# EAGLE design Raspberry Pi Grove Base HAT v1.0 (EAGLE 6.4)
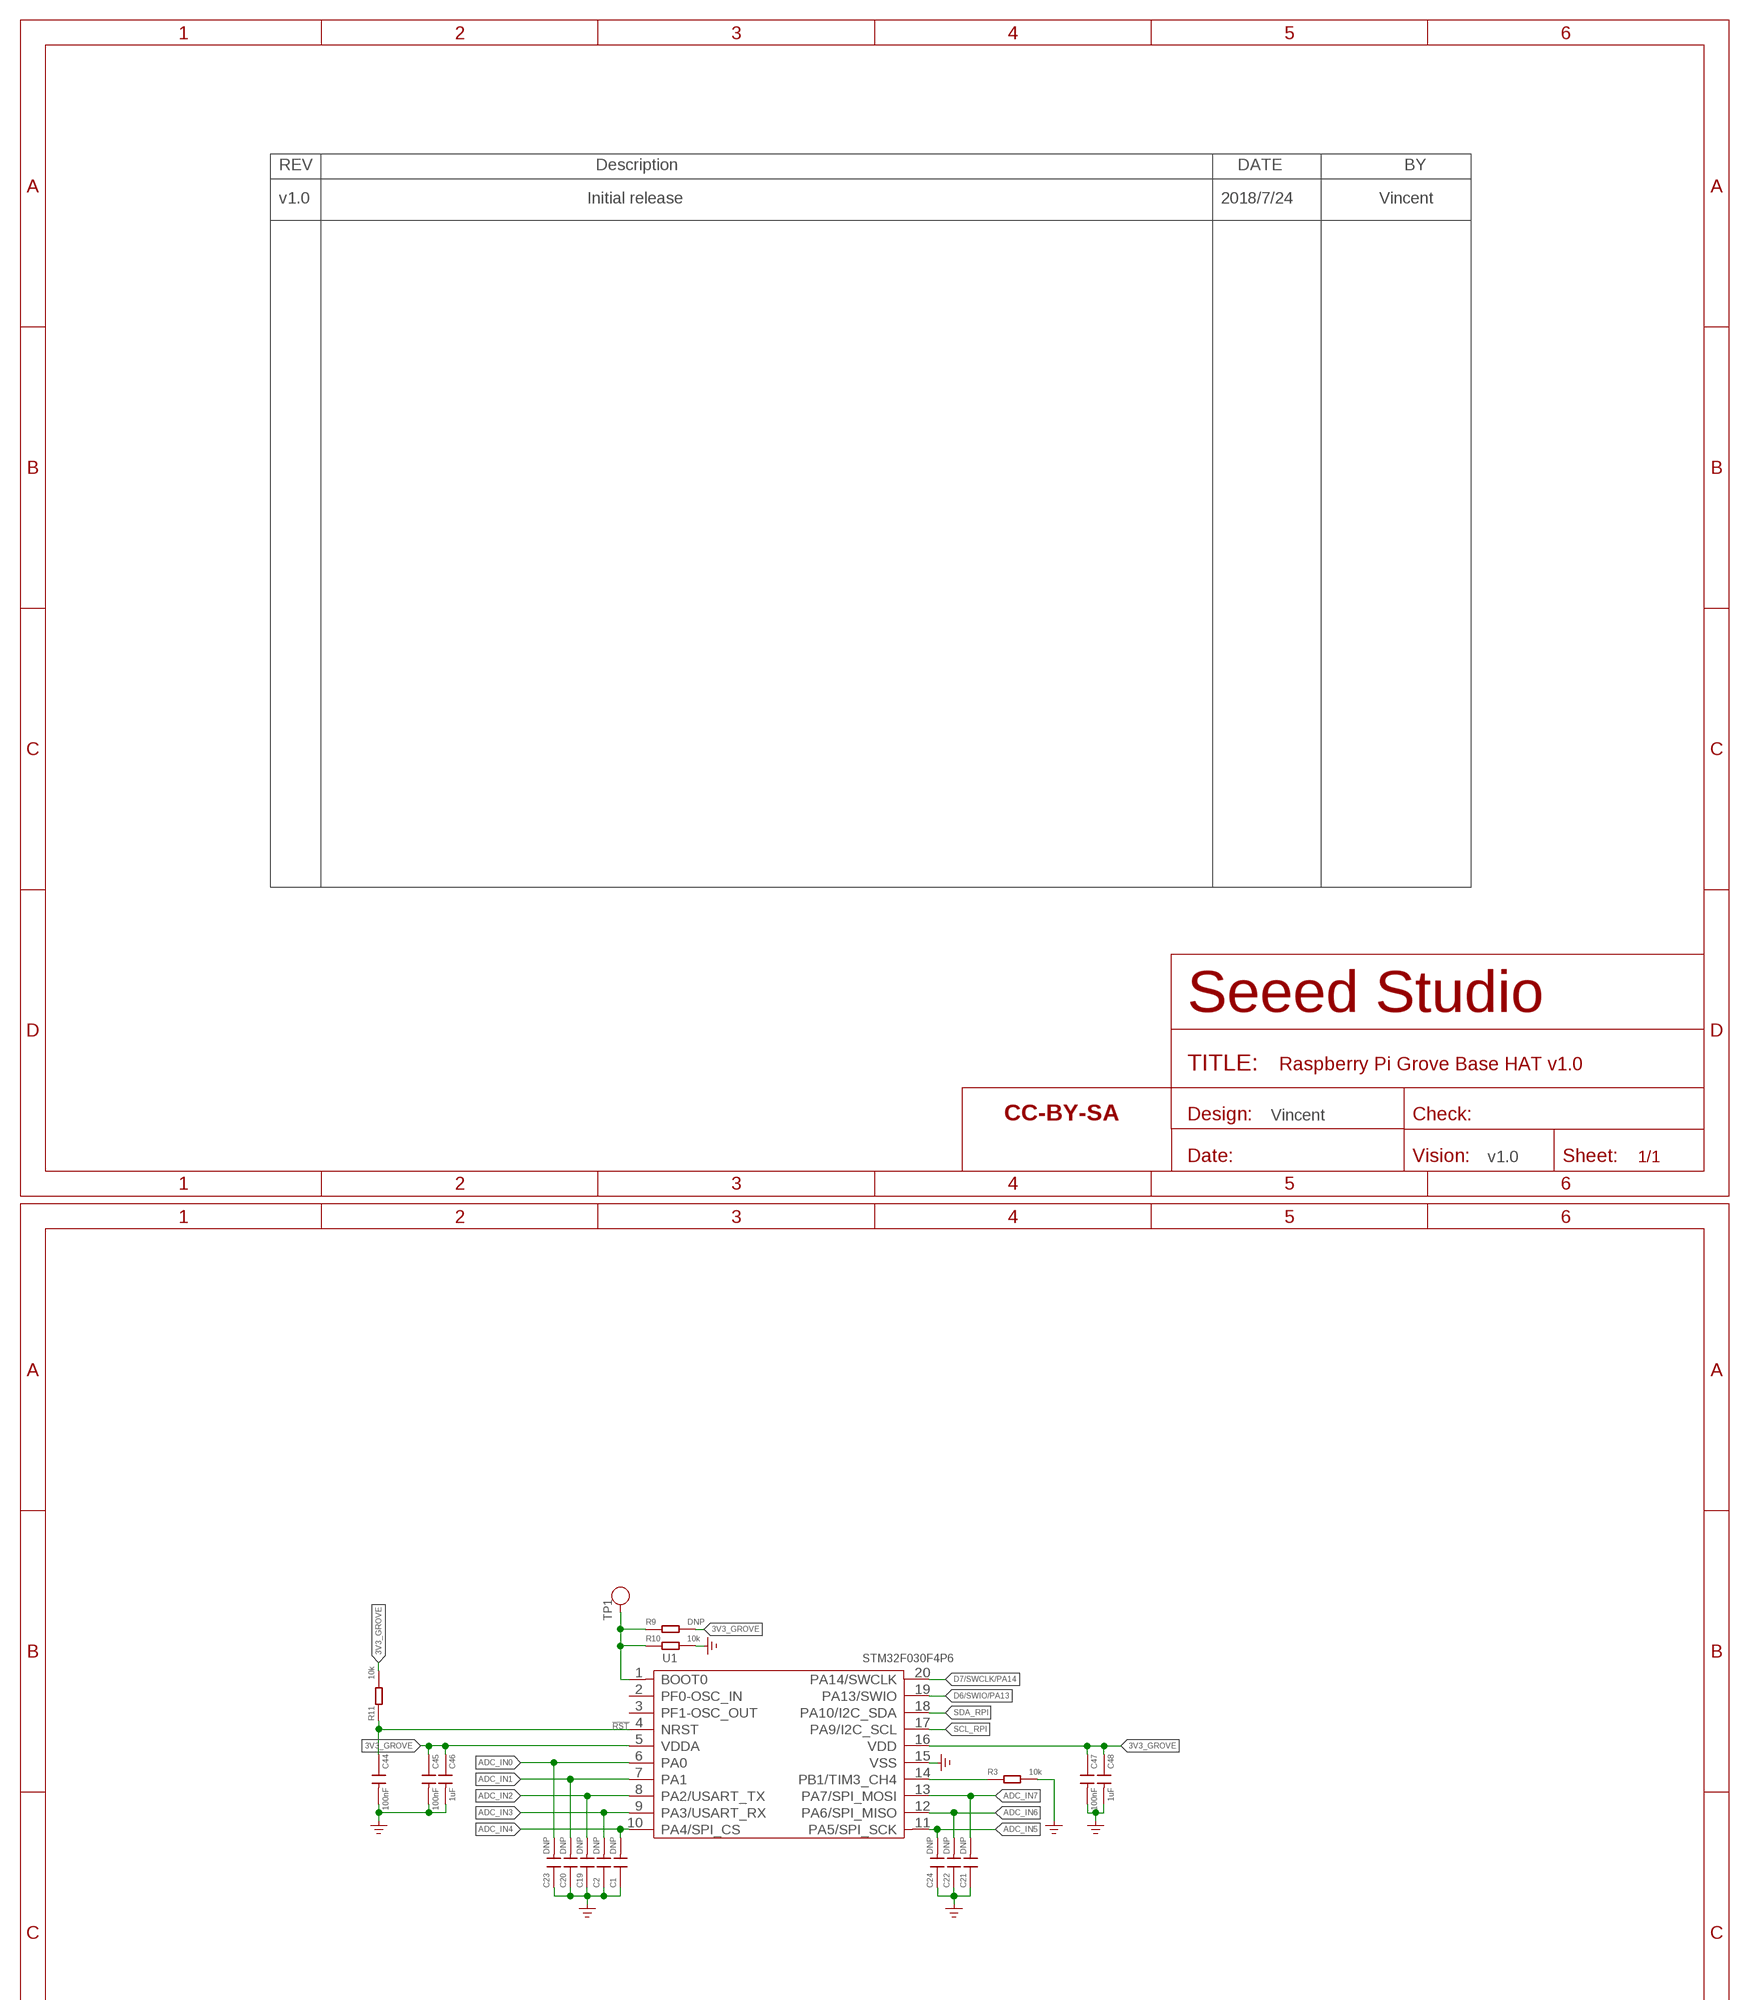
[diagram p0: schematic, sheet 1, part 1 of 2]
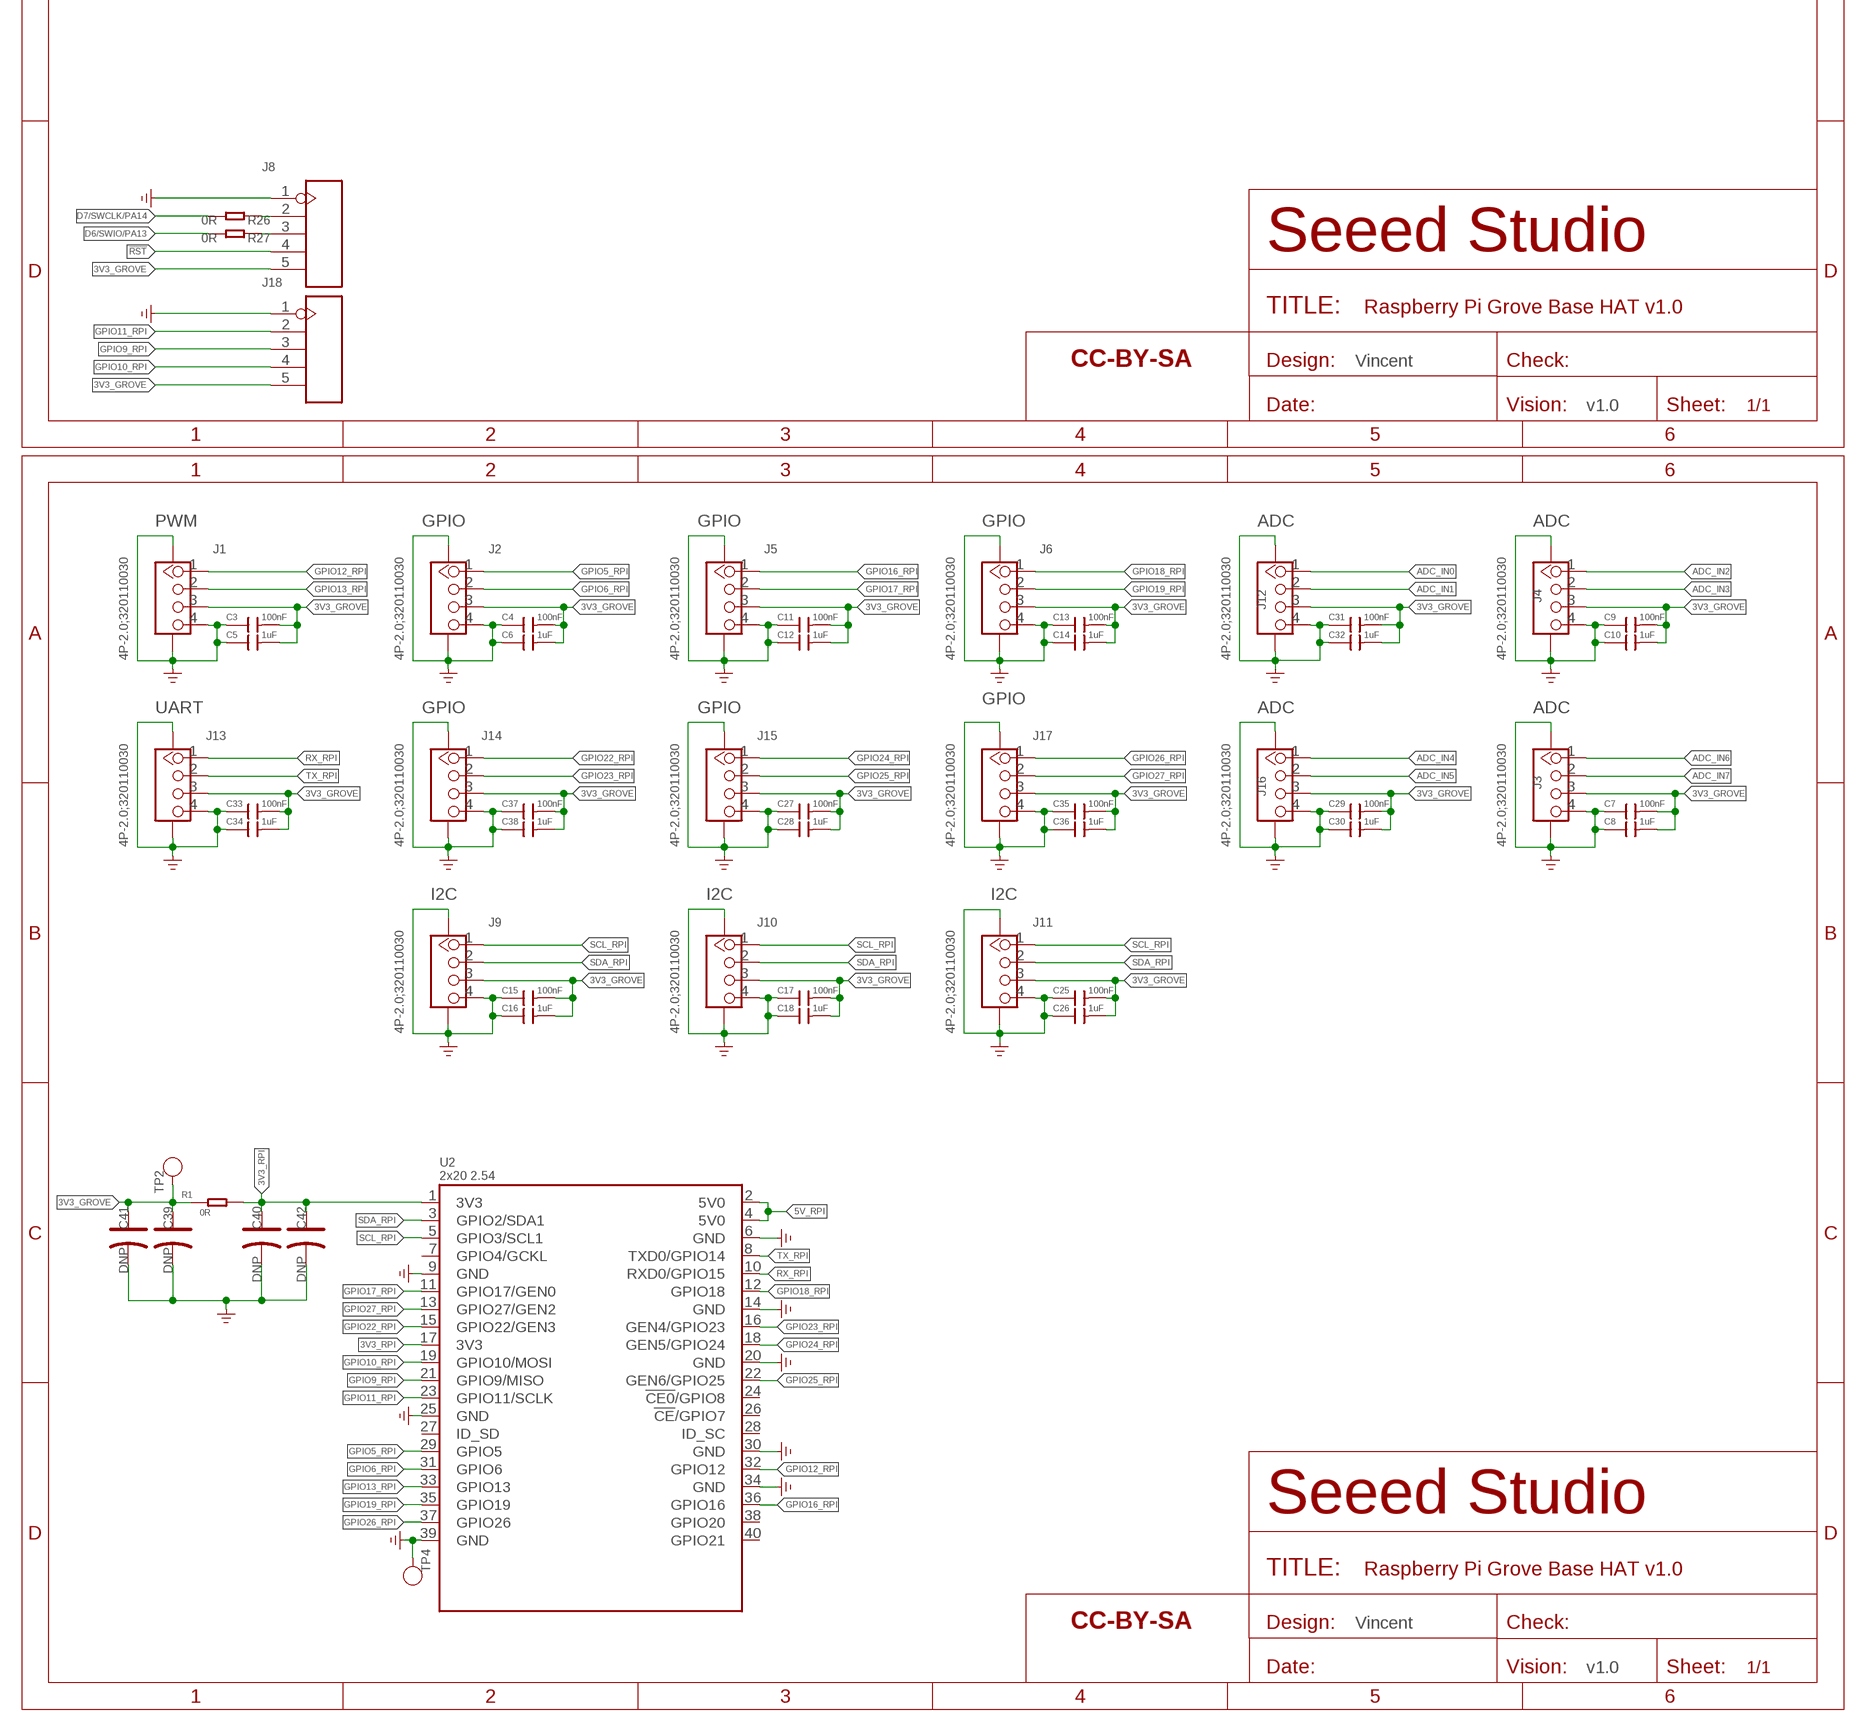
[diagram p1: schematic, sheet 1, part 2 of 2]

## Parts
C1  DNP  C-0603  [C0603]
C2  DNP  C-0603  [C0603]
C3  100nF  C-0603  [C0603]
C4  100nF  C-0603  [C0603]
C5  1uF  C-0603  [C0603]
C6  1uF  C-0603  [C0603]
C7  100nF  C-0603  [C0603]
C8  1uF  C-0603  [C0603]
C9  100nF  C-0603  [C0603]
C10  1uF  C-0603  [C0603]
C11  100nF  C-0603  [C0603]
C12  1uF  C-0603  [C0603]
C13  100nF  C-0603  [C0603]
C14  1uF  C-0603  [C0603]
C15  100nF  C-0603  [C0603]
C16  1uF  C-0603  [C0603]
C17  100nF  C-0603  [C0603]
C18  1uF  C-0603  [C0603]
C19  DNP  C-0603  [C0603]
C20  DNP  C-0603  [C0603]
C21  DNP  C-0603  [C0603]
C22  DNP  C-0603  [C0603]
C23  DNP  C-0603  [C0603]
C24  DNP  C-0603  [C0603]
C25  100nF  C-0603  [C0603]
C26  1uF  C-0603  [C0603]
C27  100nF  C-0603  [C0603]
C28  1uF  C-0603  [C0603]
C29  100nF  C-0603  [C0603]
C30  1uF  C-0603  [C0603]
C31  100nF  C-0603  [C0603]
C32  1uF  C-0603  [C0603]
C33  100nF  C-0603  [C0603]
C34  1uF  C-0603  [C0603]
C35  100nF  C-0603  [C0603]
C36  1uF  C-0603  [C0603]
C37  100nF  C-0603  [C0603]
C38  1uF  C-0603  [C0603]
C39  DNP  CAP-POLAR-AVX-B  [AVX-B]
C40  DNP  CAP-POLAR-AVX-B  [AVX-B]
C41  DNP  CAP-POLAR-AVX-B  [AVX-B]
C42  DNP  CAP-POLAR-AVX-B  [AVX-B]
C44  100nF  C-0603  [C0603]
C45  100nF  C-0603  [C0603]
C46  1uF  C-0603  [C0603]
C47  100nF  C-0603  [C0603]
C48  1uF  C-0603  [C0603]
FR  SEEEDSTUDIO-OPEN-SCH-FRAME  [SEEEDSTUDIO-PCB-FRAME]
FR1  SEEEDSTUDIO-OPEN-SCH-FRAME  [SEEEDSTUDIO-PCB-FRAME]
FR2  SEEEDSTUDIO-OPEN-SCH-FRAME  [SEEEDSTUDIO-PCB-FRAME]
J1  4P-2.0;320110030  GROVE-CONNECTOR-SMD'DD'  [HW4-SMD-2.0]
J2  4P-2.0;320110030  GROVE-CONNECTOR-SMD'DD'  [HW4-SMD-2.0]
J3  4P-2.0;320110030  GROVE-CONNECTOR-SMD'DD'  [HW4-SMD-2.0]
J4  4P-2.0;320110030  GROVE-CONNECTOR-SMD'DD'  [HW4-SMD-2.0]
J5  4P-2.0;320110030  GROVE-CONNECTOR-SMD'DD'  [HW4-SMD-2.0]
J6  4P-2.0;320110030  GROVE-CONNECTOR-SMD'DD'  [HW4-SMD-2.0]
J8  HEADER-5P-2.54  [H5-2.54]
J9  4P-2.0;320110030  GROVE-CONNECTOR-SMD'DD'  [HW4-SMD-2.0]
J10  4P-2.0;320110030  GROVE-CONNECTOR-SMD'DD'  [HW4-SMD-2.0]
J11  4P-2.0;320110030  GROVE-CONNECTOR-SMD'DD'  [HW4-SMD-2.0]
J12  4P-2.0;320110030  GROVE-CONNECTOR-SMD'DD'  [HW4-SMD-2.0]
J13  4P-2.0;320110030  GROVE-CONNECTOR-SMD'DD'  [HW4-SMD-2.0]
J14  4P-2.0;320110030  GROVE-CONNECTOR-SMD'DD'  [HW4-SMD-2.0]
J15  4P-2.0;320110030  GROVE-CONNECTOR-SMD'DD'  [HW4-SMD-2.0]
J16  4P-2.0;320110030  GROVE-CONNECTOR-SMD'DD'  [HW4-SMD-2.0]
J17  4P-2.0;320110030  GROVE-CONNECTOR-SMD'DD'  [HW4-SMD-2.0]
J18  HEADER-5P-2.54  [H5-2.54]
R1  0R  R-0805  [R0805]
R3  10k  R-0603  [R0603]
R9  DNP  R-0603  [R0603]
R10  10k  R-0603  [R0603]
R11  10k  R-0603  [R0603]
R26  0R  R-0603  [R0603]
R27  0R  R-0603  [R0603]
TP1  TEST-POINT'4545'  [TP-D45MIL@1]
TP2  TEST-POINT'4545'  [TP-D45MIL@1]
TP4  TEST-POINT'4545'  [TP-D45MIL@1]
U1  STM32F030F4P6  MCU-STM32F030  [TSSOP20-0.65-6.5X4.4MM]
U2  2x20 2.54  RPI-ZERO-65X56  [RASPI_BOARD_B+HAT_DF_CF]

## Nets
3V3_GROVE: C3.2 C4.2 C5.2 C6.2 C7.2 C8.2 C9.2 C10.2 C11.2 C12.2 C13.2 C14.2 C15.2 C16.2 C17.2 C18.2 C25.2 C26.2 C27.2 C28.2 C29.2 C30.2 C31.2 C32.2 C33.2 C34.2 C35.2 C36.2 C37.2 C38.2 C39.+ C41.+ C45.1 C46.1 C47.1 C48.1 J1.3 J2.3 J3.3 J4.3 J5.3 J6.3 J8.5 J9.3 J10.3 J11.3 J12.3 J13.3 J14.3 J15.3 J16.3 J17.3 J18.5 R1.1 R9.2 R11.2 TP2.T U1.5(VDDA) U1.16(VDD)
3V3_RPI: C40.+ C42.+ R1.2 U2.1(3V3) U2.17(3V3)
5V_RPI: U2.2(5V0) U2.4(5V0)
!RST: C44.1 J8.4 R11.1 U1.4(NRST)
ADC_IN0: C23.2 J12.1 U1.6(PA0)
ADC_IN1: C20.2 J12.2 U1.7(PA1)
ADC_IN2: C19.2 J4.1 U1.8(PA2/USART_TX)
ADC_IN3: C2.2 J4.2 U1.9(PA3/USART_RX)
ADC_IN4: C1.2 J16.1 U1.10(PA4/SPI_CS)
ADC_IN5: C24.2 J16.2 U1.11(PA5/SPI_SCK)
ADC_IN6: C22.2 J3.1 U1.12(PA6/SPI_MISO)
ADC_IN7: C21.2 J3.2 U1.13(PA7/SPI_MOSI)
D6/SWIO/PA13: R27.2 U1.19(PA13/SWIO)
D7/SWCLK/PA14: R26.2 U1.20(PA14/SWCLK)
GND: C1.1 C2.1 C3.1 C4.1 C5.1 C6.1 C7.1 C8.1 C9.1 C10.1 C11.1 C12.1 C13.1 C14.1 C15.1 C16.1 C17.1 C18.1 C19.1 C20.1 C21.1 C22.1 C23.1 C24.1 C25.1 C26.1 C27.1 C28.1 C29.1 C30.1 C31.1 C32.1 C33.1 C34.1 C35.1 C36.1 C37.1 C38.1 C39.- C40.- C41.- C42.- C44.2 C45.2 C46.2 C47.2 C48.2 J1.4 J1.SS1 J1.SS2 J2.4 J2.SS1 J2.SS2 J3.4 J3.SS1 J3.SS2 J4.4 J4.SS1 J4.SS2 J5.4 J5.SS1 J5.SS2 J6.4 J6.SS1 J6.SS2 J8.1 J9.4 J9.SS1 J9.SS2 J10.4 J10.SS1 J10.SS2 J11.4 J11.SS1 J11.SS2 J12.4 J12.SS1 J12.SS2 J13.4 J13.SS1 J13.SS2 J14.4 J14.SS1 J14.SS2 J15.4 J15.SS1 J15.SS2 J16.4 J16.SS1 J16.SS2 J17.4 J17.SS1 J17.SS2 J18.1 R3.2 R10.2 TP4.T U1.15(VSS) U2.6(GND) U2.9(GND) U2.14(GND) U2.20(GND) U2.25(GND) U2.30(GND) U2.34(GND) U2.39(GND) ; supply symbol labelled GND_POWER
GPIO5_RPI: J2.1 U2.29(GPIO5)
GPIO6_RPI: J2.2 U2.31(GPIO6)
GPIO9_RPI: J18.3 U2.21(GPIO9/MISO)
GPIO10_RPI: J18.4 U2.19(GPIO10/MOSI)
GPIO11_RPI: J18.2 U2.23(GPIO11/SCLK)
GPIO12_RPI: J1.1 U2.32(GPIO12)
GPIO13_RPI: J1.2 U2.33(GPIO13)
GPIO16_RPI: J5.1 U2.36(GPIO16)
GPIO17_RPI: J5.2 U2.11(GPIO17/GEN0)
GPIO18_RPI: J6.1 U2.12(GPIO18)
GPIO19_RPI: J6.2 U2.35(GPIO19)
GPIO22_RPI: J14.1 U2.15(GPIO22/GEN3)
GPIO23_RPI: J14.2 U2.16(GEN4/GPIO23)
GPIO24_RPI: J15.1 U2.18(GEN5/GPIO24)
GPIO25_RPI: J15.2 U2.22(GEN6/GPIO25)
GPIO26_RPI: J17.1 U2.37(GPIO26)
GPIO27_RPI: J17.2 U2.13(GPIO27/GEN2)
N$1: R3.1 U1.14(PB1/TIM3_CH4)
N$2: J8.2 R26.1
N$3: J8.3 R27.1
N$8: R9.1 R10.1 TP1.T U1.1(BOOT0)
RX_RPI: J13.1 U2.10(RXD0/GPIO15)
SCL_RPI: J9.1 J10.1 J11.1 U1.17(PA9/I2C_SCL) U2.5(GPIO3/SCL1)
SDA_RPI: J9.2 J10.2 J11.2 U1.18(PA10/I2C_SDA) U2.3(GPIO2/SDA1)
TX_RPI: J13.2 U2.8(TXD0/GPIO14)
Unconnected: U1.2(PF0-OSC_IN) U1.3(PF1-OSC_OUT) U2.7(GPIO4/GCKL) U2.24(!CE0!/GPIO8) U2.26(!CE!/GPIO7) U2.27(ID_SD) U2.28(ID_SC) U2.38(GPIO20) U2.40(GPIO21)

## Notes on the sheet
- v1.0 | Initial release | 2018/7/24 | Vincent
- Vincent
- v1.0
- Vincent
- v1.0
- PWM | GPIO | GPIO | GPIO | ADC | ADC
- GPIO
- UART | GPIO | GPIO | ADC | ADC
- I2C | I2C | I2C
- Vincent
- v1.0

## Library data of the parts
C1-C38 C44-C48 = Discrete-small:C*: Ceramic Capacitors
C39-C42 = Discrete-new:CAP-POLAR: Electrolytic Capacitors,Tantalum Capacitors and Super Capacitors
FR FR1 FR2 = moudle-new:SEEEDSTUDIO-OPEN-SCH-FRAME
J1-J6 J9-J17 = Connector-new:GROVE-CONNECTOR-SMD: 4P-SMD-2.0:320110030;4P-SMD-2.0-90D:320110032
J8 J18 = Connector-new:HEADER-5P
R1 R3 R9-R11 R26 R27 = Discrete-small:R*
TP1 TP2 TP4 = Discrete-new:TEST-POINT; PARTNO: DNP
U1 = G2:MCU-STM32F030
U2 = IC-new:RPI-ZERO

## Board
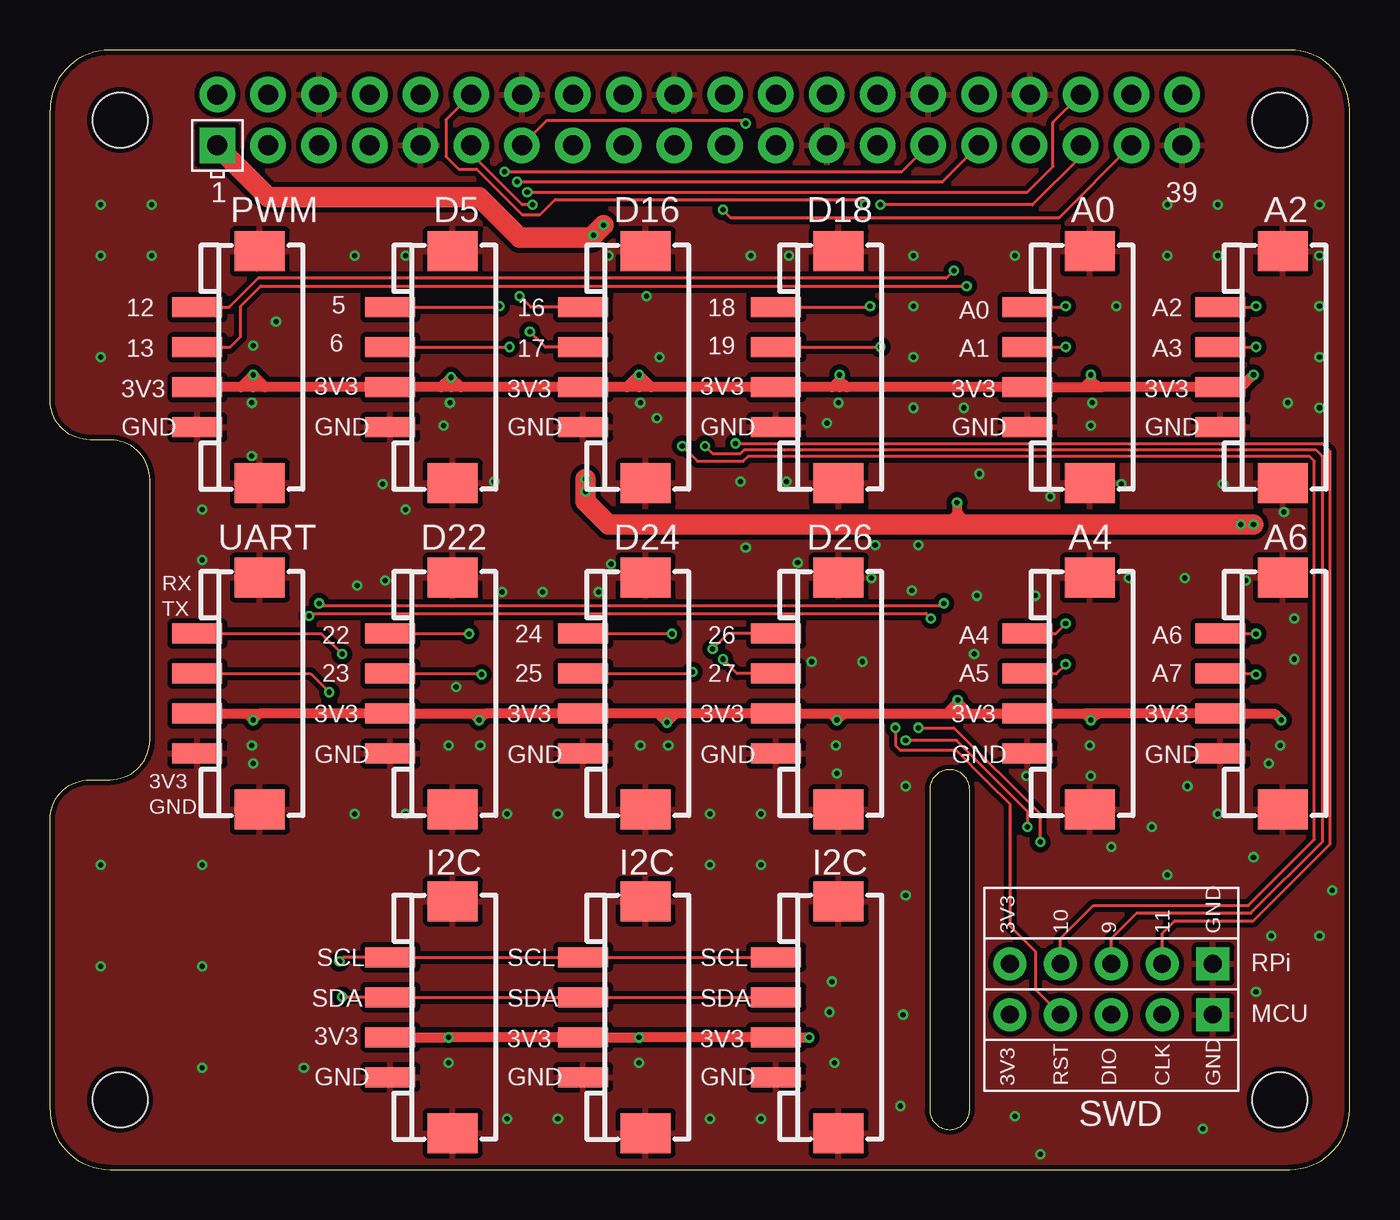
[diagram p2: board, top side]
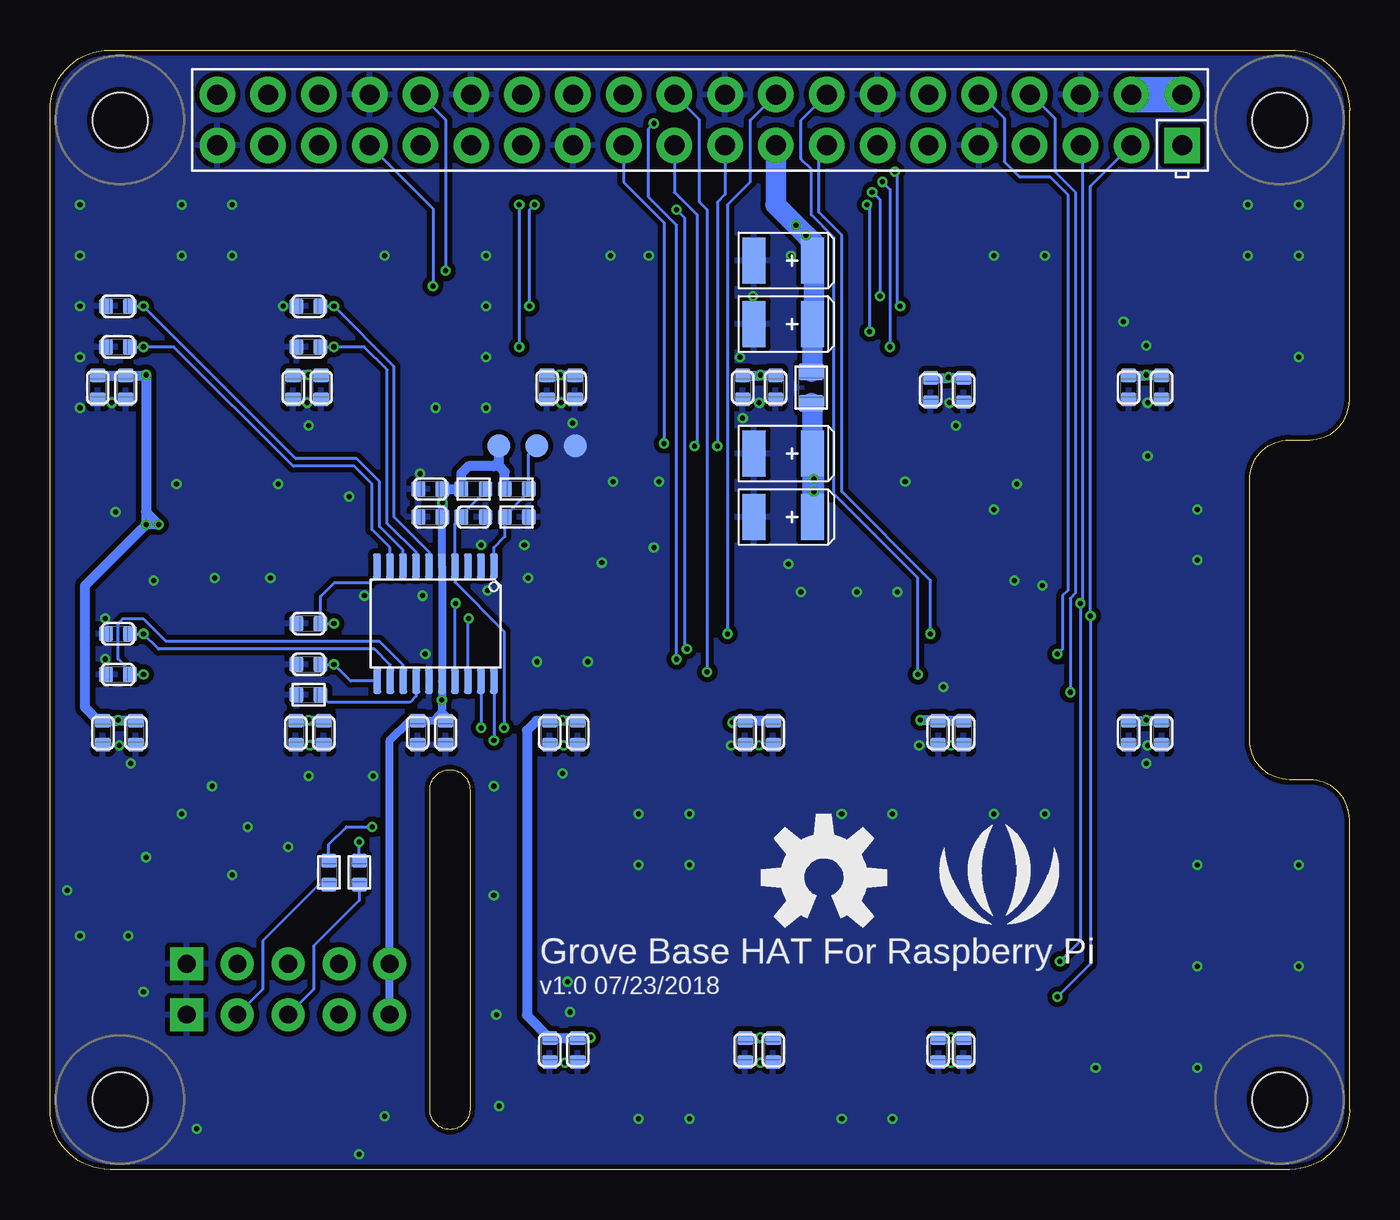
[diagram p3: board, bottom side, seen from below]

Size 65 x 56 mm. Coordinates in mm from the lower left corner, seen from the top.
Copper layers (1*16): Top 0.035mm / dielectric 1.5mm / Bottom 0.035mm
Design rules "SeeedStudio_2layer_DRU_no_angle_20140221 *": minimum track width 1mil, minimum drill 10mil, track to track 6mil, track to pad 6mil, pad to pad 6mil, via to via 6mil, smd to smd 0mil, copper to edge 10mil, drill to drill 10mil, minimum pad ring 4mil, minimum via ring 4mil, stop-mask expansion 2mil, vias tented up to drill 25mil, thermal gap 10mil

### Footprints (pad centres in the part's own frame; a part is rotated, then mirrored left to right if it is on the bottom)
C0603 = smd 0.762 x 0.696: 1 0,0.602; 2 0,-0.602
AVX-B = smd 1.143 x 2.286: + 1.46,0; - -1.46,0
HW4-SMD-2.0 = smd 1 x 2.5: 1 -3,0; 2 -1,0; 3 1,0; 4 3,0 | smd 2 x 2.5: SS1 -5.8,3.123; SS2 5.8,3.123
H5-2.54 = drill 0.889 pad 1.651 square: 1 0,5.08 | drill 0.889 pad 1.651: 2 0,2.54; 3 0,0; 4 0,-2.54; 5 0,-5.08
R0805 = smd 0.819 x 1.27: 1 -0.79,0; 2 0.79,0
R0603 = smd 0.762 x 0.696: 1 0,0.602; 2 0,-0.602
TP-D45MIL@1 = smd 1.143 x 1.143: T 0,0
TSSOP20-0.65-6.5X4.4MM = smd 0.394 x 1.27: 1 -2.925,-2.875; 2 -2.275,-2.875; 3 -1.625,-2.875; 4 -0.975,-2.875; 5 -0.325,-2.875; 6 0.325,-2.875; 7 0.975,-2.875; 8 1.625,-2.875; 9 2.275,-2.875; 10 2.925,-2.875; 11 2.91,2.875; 12 2.26,2.875; 13 1.61,2.875; 14 0.96,2.875; 15 0.325,2.875; 16 -0.325,2.875; 17 -0.975,2.875; 18 -1.625,2.875; 19 -2.275,2.875; 20 -2.925,2.875
RASPI_BOARD_B+HAT_DF_CF = drill 1 pad 1.778 square: 1 8.37,51.23 | drill 1 pad 1.778: 2 8.37,53.77; 3 10.91,51.23; 4 10.91,53.77; 5 13.45,51.23; 6 13.45,53.77; 7 15.99,51.23; 8 15.99,53.77; 9 18.53,51.23; 10 18.53,53.77; 11 21.07,51.23; 12 21.07,53.77; 13 23.61,51.23; 14 23.61,53.77; 15 26.15,51.23; 16 26.15,53.77; 17 28.69,51.23; 18 28.69,53.77; 19 31.23,51.23; 20 31.23,53.77; 21 33.77,51.23; 22 33.77,53.77; 23 36.31,51.23; 24 36.31,53.77; 25 38.85,51.23; 26 38.85,53.77; 27 41.39,51.23; 28 41.39,53.77; 29 43.93,51.23; 30 43.93,53.77; 31 46.47,51.23; 32 46.47,53.77; 33 49.01,51.23; 34 49.01,53.77; 35 51.55,51.23; 36 51.55,53.77; 37 54.09,51.23; 38 54.09,53.77; 39 56.63,51.23; 40 56.63,53.77 | hole 2.75: 3.5,3.5; 3.5,52.5; 61.5,3.5; 61.5,52.5

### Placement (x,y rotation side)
C1  52.07,27.3 90 bottom
C2  61.59,41.15 90 bottom
C3  9.4,39.12 180 bottom
C4  19.3,38.99 180 bottom
C5  11.05,39.12 180 bottom
C6  20.95,38.99 180 bottom
C7  60.71,21.84 180 bottom
C8  62.36,21.84 180 bottom
C9  62.61,39.12 180 bottom
C10  61.21,39.12 180 bottom
C11  28.7,39.12 180 bottom
C12  30.35,39.12 180 bottom
C13  38.73,39.12 180 bottom
C14  40.13,39.12 180 bottom
C15  19.3,5.97 180 bottom
C16  20.57,5.97 180 bottom
C17  28.83,5.97 180 bottom
C18  30.23,5.97 180 bottom
C19  61.59,43.18 90 bottom
C20  52.07,41.15 90 bottom
C21  61.59,24.77 90 bottom
C22  61.59,26.8 90 bottom
C23  52.07,43.18 90 bottom
C24  52.07,25.27 90 bottom
C25  38.61,5.97 180 bottom
C26  40.01,5.97 180 bottom
C27  30.23,21.84 180 bottom
C28  28.83,21.84 180 bottom
C29  51.31,21.84 180 bottom
C30  52.7,21.84 180 bottom
C31  51.44,39.12 180 bottom
C32  52.83,39.12 180 bottom
C33  11.05,21.84 180 bottom
C34  9.4,21.84 180 bottom
C35  38.61,21.84 180 bottom
C36  40.01,21.84 180 bottom
C37  20.57,21.84 180 bottom
C38  19.3,21.84 180 bottom
C39  28.32,35.81 0 bottom
C40  28.32,42.29 0 bottom
C41  28.32,32.64 0 bottom
C42  28.32,45.47 0 bottom
C44  43.81,32.64 90 bottom
C45  45.97,32.64 270 bottom
C46  45.97,34.04 270 bottom
C47  45.21,21.84 0 bottom
C48  46.61,21.84 0 bottom
FR  not placed on the board
FR1  not placed on the board
FR2  not placed on the board
J1  7.37,40.13 270 top
J2  17.02,40.13 270 top
J3  58.55,23.81 270 top
J4  58.55,40.13 270 top
J5  26.67,40.13 270 top
J6  36.32,40.13 270 top
J8  53.09,7.75 270 top
J9  17.02,7.62 270 top
J10  26.67,7.62 270 top
J11  36.32,7.62 270 top
J12  48.9,40.13 270 top
J13  7.37,23.81 270 top
J14  17.02,23.81 270 top
J15  26.67,23.81 270 top
J16  48.9,23.81 270 top
J17  36.32,23.81 270 top
J18  53.09,10.29 270 top
R1  26.92,39.12 90 bottom
R3  52.07,23.75 270 bottom
R9  41.66,34.04 270 bottom
R10  41.66,32.64 90 bottom
R11  43.81,34.04 270 bottom
R26  51.05,14.86 180 bottom
R27  49.53,14.86 180 bottom
TP1  40.64,36.2 90 bottom
TP2  42.55,36.2 0 bottom
TP4  38.73,36.2 0 bottom
U1  45.72,27.3 180 bottom
U2  0,0 0 top
U$46  [SEEED-SILK-280*268MIL]  17.53,13.97 0 bottom
U$47  [OSHW_FILLX250_NOTEXT]  26.29,14.61 0 bottom

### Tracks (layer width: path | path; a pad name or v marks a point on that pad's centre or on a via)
3V3_GROVE  (via drill 0.25 pad 0.51)
  Top 0.406: v45.4,23.5 45.4,22.88 45.47,22.81 | 44.96,22.81 44.96,22.99 45.47,23.5 45.47,23.37 45.97,22.86
  Top 0.508: v60.2,39.75 59.58,39.13 J4.3 52.44,39.13 52.07,39.5 | v61.59,22.48 61.26,22.81 J3.3 52.07,22.81 | 52.07,22.81 51.74,22.81 v52.07,22.48 | v52.07,22.48 52.07,22.73 | 52.07,22.73 52.07,22.81 | v52.07,22.48 52.32,22.73 | 39.04,22.81 J17.3 31.32,22.81 | 39.04,22.81 39.37,22.81 | 39.37,22.81 39.7,22.81 | v39.37,22.48 39.37,22.81 | 39.04,22.81 v39.37,22.48 | 39.7,22.81 v39.37,22.48 | 39.86,39.13 J12.3 51.7,39.13 | 39.86,39.13 39.5,39.13 | 39.5,39.13 39.13,39.13 | 39.13,39.13 J6.3 30.08,39.13 | v39.5,39.75 39.5,39.5 | 39.5,39.5 39.5,39.13 | 39.13,39.13 39.5,39.5 | 39.86,39.13 39.5,39.5 | 51.7,39.13 52.07,39.13 | 52.07,39.13 52.59,39.13 | v52.07,39.75 52.07,39.5 | 52.07,39.5 52.07,39.13 | 51.7,39.13 52.07,39.5 | 30.08,39.13 29.46,39.13 | 29.46,39.13 28.84,39.13 | 28.84,39.13 J5.3 20.56,39.13 | v29.46,39.75 29.46,39.13 | 28.84,39.13 v29.46,39.75 | 30.08,39.13 v29.46,39.75 | 20.56,39.13 20.08,39.13 | 20.08,39.13 19.57,39.13 | 19.57,39.13 17.03,39.13 | 17.03,39.13 17.02,39.12 J2.3 | 20.08,39.13 20.08,39.61 v20.07,39.62 | 19.57,39.13 v20.07,39.62 | 20.56,39.13 v20.07,39.62 | 17.03,39.13 10.78,39.13 | 10.78,39.13 10.16,39.13 | 10.16,39.13 9.54,39.13 | 9.54,39.13 J1.3 | v10.16,39.75 10.16,39.13 | 9.54,39.13 v10.16,39.75 | 10.78,39.13 v10.16,39.75 | 31.32,22.81 30.86,22.81 | 30.86,22.81 30.4,22.81 | 30.4,22.81 J15.3 21.8,22.81 | v30.86,22.35 30.86,22.81 | 30.4,22.81 v30.86,22.35 | 31.32,22.81 v30.86,22.35 | 21.8,22.81 v21.46,22.48 21.13,22.81 | 21.13,22.81 J14.3 10.49,22.81 | 21.13,22.81 21.8,22.81 | 10.49,22.81 v10.16,22.48 9.83,22.81 | J13.3 9.83,22.81 | 9.83,22.81 10.49,22.81 | v37.97,6.6 37.96,6.62 J11.3 29.48,6.62 v29.46,6.6 29.45,6.62 J10.3 19.95,6.62 v19.94,6.6 19.92,6.62 J9.3
  Top 0.508: 52.07,22.73 51.99,22.81 J16.3 45.47,22.81 44.96,22.81 39.7,22.81 | v45.37,33.37 45.37,32.16 | 44.58,32.26 44.7,32.13 45.34,32.77 45.47,32.77 45.97,32.26
  Top 1.016: v60.2,32.26 44.58,32.26 27.94,32.26 26.8,33.4 v26.8,34.54
  Bottom 0.406: C45.1 45.4,32.62 U1.5 U1.16 45.4,22.99 | C47.1 45.4,22.63 45.4,22.85 45.09,22.54 | C47.1 45.82,22.45 | 45.82,22.45 C48.1 47.02,22.45 48.01,21.46 J18.5 J8.5 | C38.2 19.3,22.35 | C28.2 28.73,22.45 | 30.87,22.36 v30.86,22.35 | 45.82,22.45 45.4,22.86 | v45.4,23.5 45.4,22.99 | 45.4,22.99 45.4,22.64 C47.1
  Bottom 0.508: 45.37,33.78 C46.1 R11.2 44.42,34.83 44.07,35.18 42.8,35.18 | 45.37,33.78 45.37,33.62 | C45.1 v45.37,33.37 45.37,33.62 | R9.2 42.26,34.89 42.55,35.18 | 42.55,35.18 42.8,35.18 | 45.37,33.62 45.34,33.66 45.34,33.75 45.37,33.78 | 42.55,35.18 42.55,35.43 | 42.8,35.18 42.55,35.43 | C9.2 C10.2 60.23,39.72 v60.2,39.75 60.2,32.89 | C32.2 52.87,39.75 v52.07,39.75 52.04,39.72 C31.2 | 60.2,32.89 v60.2,32.26 | C7.2 61.56,22.45 v61.59,22.48 61.63,22.45 C8.2 62.58,22.45 63.25,23.11 63.25,29.21 v60.2,32.26 | C29.2 52.04,22.45 v52.07,22.48 52.1,22.45 C30.2 | C35.2 39.34,22.45 v39.37,22.48 39.4,22.45 C36.2 40.67,22.45 41.15,21.97 41.15,7.71 C26.2 C25.2 38.01,6.57 v37.97,6.6 | C14.2 39.53,39.72 v39.5,39.75 39.46,39.72 C13.2 | C12.2 29.5,39.72 v29.46,39.75 29.43,39.72 C11.2 | C4.2 20.03,39.59 v20.07,39.62 20.1,39.59 C6.2 | C5.2 10.19,39.72 v10.16,39.75 10.13,39.72 C3.2 | v30.86,22.35 30.77,22.45 C27.2 C28.2 | v21.46,22.48 20.61,22.48 C37.2 C38.2 | C34.2 10.13,22.45 v10.16,22.48 10.19,22.45 C33.2 | C18.2 29.5,6.57 v29.46,6.6 29.43,6.57 C17.2 | C16.2 19.97,6.57 v19.94,6.6 19.91,6.57 C15.2 | v60.2,32.26 v59.56,32.26 60.2,32.89 | 42.55,35.43 TP2.T
  Bottom 1.016: R1.1 26.86,38.26 C39.+ C41.+ 26.8,32.7 v26.8,33.91 v26.8,34.54 26.8,35.81
3V3_RPI  (via drill 0.25 pad 0.51)
  Top 1.016: U2.1 8.37,51.19 10.92,48.64 21.46,48.64 23.5,46.61 27.05,46.61 v27.18,46.74 v27.69,47.24
  Bottom 1.016: U2.17 28.69,48.27 28.7,48.26 v27.18,46.74 26.8,46.35 26.8,45.53 | 26.8,45.53 26.8,42.35 C40.+ 26.86,39.97 R1.2 | 26.8,45.53 C42.+
5V_RPI
  Bottom 1.778: U2.2 U2.4
!RST  (via drill 0.25 pad 0.51)
  Top 0.152: v42.29,22.1 42.29,21.21 42.55,20.95 45.33,20.95 46.86,19.42 46.87,19.42 48.01,18.29 48.01,12.19 49.28,10.92 49.28,9.02 J8.4
  Bottom 0.152: R11.1 43.21,33.94 44.42,32.74 C44.1 44.74,32.31 U1.4 44.74,29.38 42.29,26.92 v42.29,22.1
ADC_IN0  (via drill 0.25 pad 0.51)
  Top 0.152: J12.1 50.75,43.13 v50.8,43.18
  Bottom 0.152: U1.6 46.05,30.89 47.79,32.64 47.79,40.17 v50.8,43.18 C23.2
ADC_IN1  (via drill 0.25 pad 0.51)
  Top 0.152: J12.2 50.78,41.13 v50.8,41.15
  Bottom 0.152: U1.7 46.7,30.88 48.13,32.32 48.13,40.01 49.28,41.15 v50.8,41.15 C20.2
ADC_IN2  (via drill 0.25 pad 0.51)
  Top 0.152: J4.1 60.28,43.13 v60.33,43.18
  Bottom 0.152: U1.8 47.34,30.99 48.51,32.16 48.51,34.42 49.66,35.56 52.7,35.56 v60.33,43.18 C19.2
ADC_IN3  (via drill 0.25 pad 0.51)
  Top 0.152: J4.2 60.31,41.13 v60.33,41.15
  Bottom 0.152: U1.9 47.99,31.1 48.9,32 48.9,34.29 49.78,35.18 52.83,35.18 58.8,41.15 v60.33,41.15 C2.2
ADC_IN4  (via drill 0.25 pad 0.51)
  Top 0.152: J16.1 50.31,26.81 v50.8,27.3
  Bottom 0.152: v50.8,27.3 C1.2 51.47,28.67 50.8,29.34 49.02,29.34 48.65,29.71 U1.10
ADC_IN5  (via drill 0.25 pad 0.51)
  Top 0.152: J16.2 50.34,24.81 v50.8,25.27
  Bottom 0.152: U1.11 49.96,24.43 v50.8,25.27 C24.2
ADC_IN6  (via drill 0.25 pad 0.51)
  Top 0.152: J3.1 60.31,26.81 v60.33,26.8
  Bottom 0.152: U1.12 47.98,25.25 48.77,26.04 59.56,26.04 v60.33,26.8 C22.2
ADC_IN7  (via drill 0.25 pad 0.51)
  Top 0.152: J3.2 60.28,24.81 v60.33,24.77
  Bottom 0.152: U1.13 47.33,25.23 48.51,26.42 59.18,26.42 60.33,27.56 61.34,27.56 61.59,27.3 61.59,25.53 60.99,24.93 C21.2 v60.33,24.77
D6/SWIO/PA13  (via drill 0.25 pad 0.51)
  Top 0.152: v43.43,22.1 45.21,22.1 49.53,17.78 v49.53,16.38
  Bottom 0.152: U1.19 43.45,22.11 v43.43,22.1 | R27.2 v49.53,16.38
D7/SWCLK/PA14  (via drill 0.25 pad 0.51)
  Top 0.152: v42.8,21.46 45.34,21.46 48.9,17.91 v48.9,17.14
  Bottom 0.152: U1.20 v42.8,21.47 v42.8,21.46 | R26.2 51.05,16.26 50.16,17.14 v48.9,17.14
GND  (via drill 0.25 pad 0.51)
  Bottom 0.508: C29.1 51.97,21.24 v52.01,21.21
  other vias: 52.13,38.35 61.91,38.35 61.53,21.21 48.83,19.68 39.31,21.21 30.92,21.21 29.53,21.21 19.94,21.21 21.53,21.21 10.1,21.21 10.1,38.35 39.43,38.35 29.53,38.35 20,38.35 10.1,35.69 19.94,5.33 29.46,5.33 39.24,5.33 2.54,48.26 5.08,48.26 2.54,45.72 5.08,45.72 17.78,45.72 27.94,45.72 43.18,45.72 48.26,45.72 55.88,45.72 58.42,45.72 63.5,45.72 63.5,43.18 63.5,40.64 43.18,43.18 43.18,40.64 43.18,38.1 45.72,38.1 2.54,40.64 10.16,41.21 29.84,43.69 53.34,43.18 63.5,38.1 38.86,37.34 7.62,33.02 17.78,33.02 7.62,30.48 10.16,20.32 2.54,15.24 2.54,10.16 7.62,10.16 7.62,15.24 12.7,5.08 7.62,5.08 22.86,2.54 25.4,2.54 33.02,2.54 35.56,2.54 48.26,2.67 35.56,15.24 33.02,15.24 25.4,17.78 22.86,17.78 15.24,17.78 17.78,17.78 58.42,48.26 55.88,48.26 35.56,17.78 33.02,17.78 38.1,25.4 40.64,25.4 63.5,48.26 60.96,20.32 58.42,17.78 19.68,37.21 30.35,37.59 16.64,34.29 56.9,19.18 39.37,19.81 42.55,3.17 42.67,7.75 42.8,13.72 42.8,19.18 39.12,9.4 38.99,7.87 16.76,29.46 15.37,29.21 11.3,42.42 46.23,25.78 46.35,28.7 49.28,28.7 52.07,37.21 20.32,24.13 27.43,28.89 24.64,28.89 22.61,28.89 28.07,30.29 37.4,30.35 41.08,29.59 43.12,28.96 62.23,27.56 62.23,25.53 49.53,0.76 61.09,11.68 55.88,14.73 60.33,8.89 55.12,17.14 57.66,2.03 53.09,16.13 60.2,15.62 63.5,11.68 64.14,13.97 52.07,19.68 53.59,34.29 61.72,32.89 53.98,29.59 59.82,29.46 56.77,29.59 36.83,34.42 34.54,34.42 46.48,34.8 34.8,31.11 22.23,34.42 15.24,45.72 36.96,45.72 35.05,45.72 30.48,40.64 41.27,31.24 43.43,31.24 58.67,34.29 50.04,33.66
  pour Bottom (isolate 0.254, rank 6): -0.64,56.52 65.41,56.52 65.41,-0.64 1.27,-0.64 1.27,-1.27 -0.64,-1.27
  pour Top (isolate 0.254, rank 6): -0.64,56.52 65.41,56.52 65.41,-0.64 -0.64,-0.64
GPIO5_RPI  (via drill 0.25 pad 0.51)
  Top 0.152: v22.73,49.91 42.61,49.91 U2.29 | J2.1 22.43,43.13 v22.48,43.18
  Bottom 0.152: v22.48,43.18 22.61,43.31 22.61,49.78 v22.73,49.91
GPIO6_RPI  (via drill 0.25 pad 0.51)
  Top 0.152: v23.37,49.4 44.64,49.4 U2.31 | J2.2 22.97,41.13 v22.99,41.15
  Bottom 0.152: v23.37,49.4 22.99,49.02 v22.99,41.15
GPIO9_RPI  (via drill 0.25 pad 0.51)
  Top 0.152: v32.77,36.2 33.15,35.81 34.54,35.81 34.73,36.01 63.31,36.01 63.63,35.69 63.63,16.38 60.07,12.83 54.36,12.83 53.09,11.56 J18.3
  Bottom 0.152: U2.21 33.77,48.88 32.64,47.75 32.64,36.32 v32.77,36.2
GPIO10_RPI  (via drill 0.25 pad 0.51)
  Top 0.152: v31.62,36.2 32.38,35.43 34.67,35.43 34.92,35.69 62.99,35.69 63.25,35.43 63.25,16.51 59.95,13.21 52.2,13.21 50.55,11.56 J18.4
  Bottom 0.152: U2.19 31.23,48.78 31.62,48.39 v31.62,36.2
GPIO11_RPI  (via drill 0.25 pad 0.51)
  Top 0.152: v34.29,36.32 63.63,36.32 64.01,35.94 64.01,16.26 60.2,12.45 56.26,12.45 55.63,11.81 J18.2
  Bottom 0.152: U2.23 36.31,49.39 34.29,47.37 v34.29,36.32
GPIO12_RPI  (via drill 0.25 pad 0.51)
  Top 0.152: v45.21,44.96 44.83,44.58 10.41,44.58 8.97,43.13 J1.1
  Bottom 0.152: U2.32 45.21,52.51 v45.21,44.96
GPIO13_RPI  (via drill 0.25 pad 0.51)
  Top 0.152: J1.2 9,41.13 9.53,41.66 9.53,43.18 10.54,44.2 v45.85,44.2
  Bottom 0.152: U2.33 45.85,48.07 v45.85,44.2
GPIO16_RPI  (via drill 0.25 pad 0.51)
  Top 0.152: v23.88,48.9 48.9,48.9 50.16,50.16 50.16,52.38 U2.36 | J5.1 24.05,43.13 v23.5,43.69
  Bottom 0.152: v23.88,48.9 23.5,48.51 v23.5,43.69
GPIO17_RPI  (via drill 0.25 pad 0.51)
  Top 0.152: v24.13,48.26 23.62,48.26 21.07,50.81 U2.11 | v24,41.91 24.32,41.59 24.38,41.53 24.78,41.13 J5.2
  Bottom 0.152: v24.13,48.26 24,48.13 v24,41.91
GPIO18_RPI  (via drill 0.25 pad 0.51)
  Top 0.152: U2.12 19.81,52.51 19.81,50.67 20.45,50.04 21.34,50.04 23.62,47.75 24.51,47.75 25.27,48.51 40.51,48.51 v40.77,48.26 | J6.1 40.97,43.13 v41.02,43.18
  Bottom 0.152: v41.02,43.18 41.02,48.01 v40.77,48.26
GPIO19_RPI  (via drill 0.25 pad 0.51)
  Top 0.152: U2.35 51.55,50.66 49.15,48.26 v41.53,48.26 | J6.2 41.51,41.13 v41.53,41.15
  Bottom 0.152: v41.53,48.26 v41.53,41.15
GPIO22_RPI  (via drill 0.25 pad 0.51)
  Top 0.152: J14.1 20.94,26.81 v20.95,26.8
  Bottom 0.152: U2.15 26.54,50.84 26.54,47.88 25.4,46.74 25.4,33.91 20.95,29.46 v20.95,26.8
GPIO23_RPI  (via drill 0.25 pad 0.51)
  Top 0.152: J14.2 21.54,24.81 v21.59,24.77
  Bottom 0.152: U2.16 27.43,52.49 27.43,50.55 26.92,50.04 26.92,47.75 25.78,46.61 25.78,33.78 21.59,29.59 v21.59,24.77
GPIO24_RPI  (via drill 0.25 pad 0.51)
  Top 0.152: J15.1 31.1,26.81 v31.11,26.8
  Bottom 0.152: U2.18 29.97,52.49 29.97,49.4 31.11,48.26 v31.11,26.8
GPIO25_RPI  (via drill 0.25 pad 0.51)
  Top 0.152: J15.2 32.05,24.81 v32.13,24.89
  Bottom 0.152: U2.22 32.51,52.51 32.51,48.39 32.13,48.01 v32.13,24.89
GPIO26_RPI  (via drill 0.25 pad 0.51)
  Top 0.152: U2.37 50.48,47.62 34.04,47.62 v33.66,48.01 | J17.1 33.92,26.81 v33.15,26.04
  Bottom 0.152: v33.66,48.01 33.27,47.62 33.27,26.16 v33.15,26.04
GPIO27_RPI  (via drill 0.25 pad 0.51)
  Top 0.152: U2.13 24.83,52.45 34.67,52.45 v34.8,52.32 | J17.2 34.37,24.81 v33.66,25.53
  Bottom 0.152: v34.8,52.32 35.05,52.07 35.05,48.64 33.66,47.24 v33.66,25.53
N$1
  Bottom 0.152: U1.14 46.68,23.68 46.99,23.37 51.09,23.37 R3.1
N$2
  Bottom 0.152: R26.1 51.53,14.26 54.36,11.43 54.36,9.02 J8.2
N$3
  Bottom 0.152: R27.1 49.53,13.46 51.82,11.18 51.82,9.02 J8.3
N$8
  Bottom 0.152: U1.1 42.8,31.12 42.26,31.66 R10.1 42.26,32.67 41.05,33.88 R9.1 41.05,35.78 TP1.T
RX_RPI  (via drill 0.25 pad 0.51)
  Top 0.152: J13.1 13.57,26.81 v14.61,25.78
  Bottom 0.152: U2.10 18.46,53.77 17.27,52.58 17.27,50.42 16.51,49.66 14.99,49.66 14.1,48.77 14.1,28.96 14.35,28.7 14.35,26.04 v14.61,25.78
SCL_RPI  (via drill 0.25 pad 0.51)
  Top 0.152: v44.7,28.32 44.58,28.19 13.59,28.19 v13.46,28.32 | J11.1 J10.1 J9.1 14.68,10.62 v14.48,10.41
  Bottom 0.152: U1.17 44.74,28.28 v44.7,28.32 | U2.5 13.34,51.12 13.34,28.45 v13.46,28.32 13.46,11.43 v14.48,10.41
SDA_RPI  (via drill 0.25 pad 0.51)
  Top 0.152: v44.07,27.56 43.81,27.81 13.08,27.81 v12.95,27.69 | v14.61,8.64 14.62,8.62 J9.2 J10.2 J11.2
  Bottom 0.152: U1.18 44.09,27.53 v44.07,27.56 | U2.3 12.95,49.19 v12.95,27.69 12.95,10.29 v14.61,8.64
TX_RPI  (via drill 0.25 pad 0.51)
  Top 0.152: J13.2 13.03,24.81 v13.97,23.88
  Bottom 0.152: U2.8 15.92,53.77 14.73,52.58 14.73,49.91 13.72,48.9 13.72,28.83 13.97,28.57 v13.97,23.88

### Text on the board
tPlace: PWM | D5 | D16 | D18 | A0 | A2 | 12 | 5 | 16 | 18 | A0 | A2 | 13 | 6 | 17 | 19 | A1 | A3 | 3V3 | 3V3 | 3V3 | 3V3 | 3V3 | 3V3 | GND | GND | GND | GND | GND | GND | UART | D22 | D24 | D26 | A4 | A6 | RX | TX | 22 | 24 | 26 | A4 | A6 | 23 | 25 | 27 | A5 | A7 | 3V3 | 3V3 | 3V3 | 3V3 | 3V3 | GND | GND | GND | GND | GND | 3V3 | GND | I2C | I2C | I2C | 3V3 | 10 | 9 | 11 | GND | SCL | SCL | SCL | RPi | SDA | SDA | SDA | MCU | 3V3 | 3V3 | 3V3 | GND | GND | GND | 3V3 | RST | DIO | CLK | GND | SWD
bPlace: Grove Base HAT For Raspberry Pi | v1.0 07/23/2018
